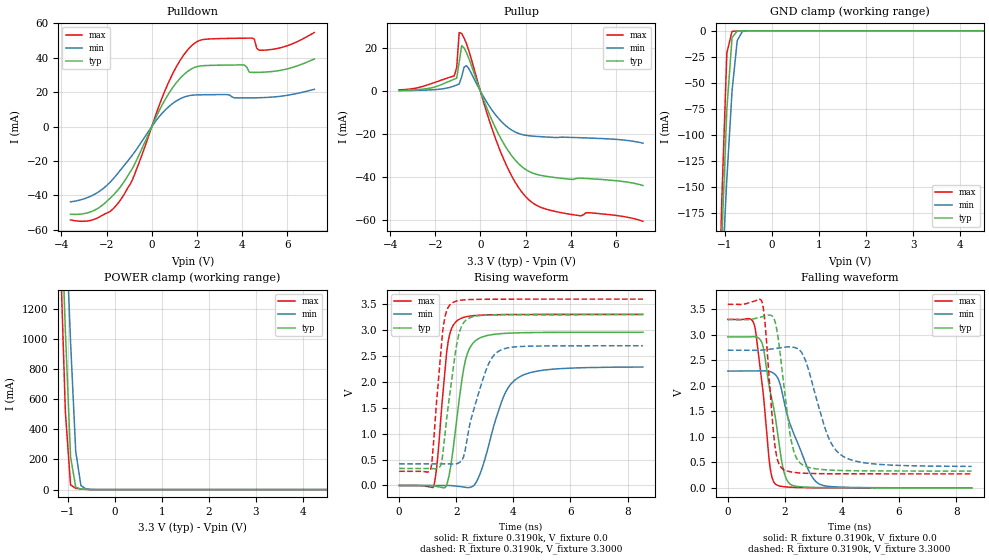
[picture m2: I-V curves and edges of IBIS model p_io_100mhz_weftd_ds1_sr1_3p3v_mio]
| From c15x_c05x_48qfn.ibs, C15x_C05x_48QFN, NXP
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[Model] p_io_100mhz_weftd_ds1_sr1_3p3v_mio
|   Model p_io_100mhz_weftd_ds1_sr1_3p3v_mio
| This model was characterised for following simulation conditions:
| External (pad) voltage:
|   - Typ: 3.3V,   - Min: 2.7V,   - Max: 3.6V
| Library cells for typ/min/max conditions are connected as defined below:
|  pad - External Pad
|  ipp_do_lv - Core Input
|  ipp_obe_lv - Output Buffer Enable
|  IOGC - NC
|  REFH3V3 - REFH3V3
|  REFL3V3 - REFL3V3
|  ZI - NC
|  abut_ncal_vddio[1] - vddio
|  abut_ncal_vddio[2] - vddio
|  abut_ncal_vddio[3] - vssio
|  abut_ncal_vddio[4] - vddio
|  abut_ncal_vddio[5] - vddio
|  abut_ncal_vddio[6] - vssio
|  abut_pcal_vddio[1] - vssio
|  abut_pcal_vddio[2] - vssio
|  abut_pcal_vddio[3] - vddio
|  abut_pcal_vddio[4] - vssio
|  abut_pcal_vddio[5] - vssio
|  abut_pcal_vddio[6] - vddio
|  ipp_do_1p8v - ipp_do_1p8v
|  ipp_dse_lv - vdd_lv
|  ipp_eftd_lv - NC
|  ipp_ina_mux_vddio - NC
|  ipp_ina_mux_vddio[0] - NC
|  ipp_ina_mux_vddio[1] - NC
|  ipp_ina_r0_vddio - NC
|  ipp_ina_r0a_vddio - NC
|  ipp_ina_r0b_vddio - NC
|  ipp_ina_r0c_vddio - NC
|  ipp_ina_r0d_vddio - NC
|  ipp_ina_r0e_vddio - NC
|  ipp_ina_r0f_vddio - NC
|  ipp_ina_r300_vddio - NC
|  ipp_ina_r300a_vddio - NC
|  ipp_ina_r300b_vddio - NC
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Model_type I/O
Polarity   Non-Inverting
Enable   Active-High
Vinl =   0.9900V
Vinh =   2.3100V
Vmeas =  1.6500V
Cref =   30.0000pF
Rref =   1.0000M
Vref =   3.3000V
C_comp   1.3824pF   1.3233pF   1.4661pF
|C_comp_pullup   0.6942pF   0.7256pF   0.6724pF
|C_comp_pulldown   0.6072pF   0.6599pF   0.5691pF
[Model Spec]
| variable   typ   min   max
Vinh   2.3100V   1.8900V   2.5200V
Vinl   0.9900V   0.8100V   1.0800V
[Temperature Range]   25.0000   0.1250k   -40.0000
[Voltage Range]   3.3000V   2.7000V   3.6000V
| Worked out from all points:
|   slope of the pulldown table from 0 to 0.495 V, typ, clamps not added: 36.8 ohm
|   slope of the pullup table from 0 to 0.495 V, typ, clamps not added: 37.8 ohm
|   GND clamp passes 1 mA (typ) near -0.75 V on its own axis
|   POWER clamp passes 1 mA (typ) near -0.55 V on its own axis
|   rising waveform, R_fixture 0.3190k, V_fixture 0.0: 20-80 % time 437ps typ, 779ps min, 310ps max; typ from 0 V to 2.96 V
|   rising waveform, R_fixture 0.3190k, V_fixture 3.3000: 20-80 % time 419ps typ, 681ps min, 295ps max; typ from 0.33 V to 3.3 V
|   falling waveform, R_fixture 0.3190k, V_fixture 0.0: 20-80 % time 516ps typ, 821ps min, 360ps max; typ from 2.96 V to 0 V
|   falling waveform, R_fixture 0.3190k, V_fixture 3.3000: 20-80 % time 404ps typ, 756ps min, 278ps max; typ from 3.3 V to 0.33 V
[Pulldown]
|Voltage   I(typ)   I(min)   I(max)
-3.6V     -50.99mA   -43.76mA   -54.26mA
-2.5V     -48.39mA   -39.11mA   -53.69mA
-1.4V     -35.22mA   -25.46mA   -42.92mA
-850mV    -24.19mA   -16.4mA    -30.69mA
800mV     20.23mA    12.14mA    27.32mA
1.35V     29.37mA    16.76mA    40.44mA
1.9V      34.45mA    18.38mA    48.57mA
4.1V      35.83mA    16.68mA    51.45mA
4.43V     31.54mA    16.72mA    51.52mA
4.65V     31.54mA    16.77mA    45.56mA
5.09V     31.78mA    16.98mA    44.58mA
7.2V      39.32mA    21.7mA     54.71mA
[Pullup]
|Voltage   I(typ)   I(min)   I(max)
-3.6V     392.3uA    235.2uA    607.2uA
-1.16V    5.571mA    2.41mA     7.094mA
-1.05V    6.017mA    2.857mA    10.99mA
-940mV    13.55mA    3.321mA    27.21mA
-830mV    21.12mA    6.673mA    26.77mA
-720mV    20.02mA    11.25mA    24.57mA
-610mV    17.72mA    11.8mA     21.82mA
820mV     -20.27mA   -12.85mA   -26.19mA
1.48V     -31.2mA    -18.62mA   -41.17mA
2.03V     -36.53mA   -20.52mA   -49.25mA
3.46V     -40.29mA   -21.47mA   -56.15mA
7.2V      -43.77mA   -24.12mA   -60.4mA
[GND_clamp]
|Voltage   I(typ)   I(min)   I(max)
-3.6V     -4.179A    -3.084A    -5.65A
-1.18V    -350.3mA   -344.8mA   -366.5mA
-1.07V    -203.5mA   -240.3mA   -165.6mA
-960mV    -75.17mA   -142.1mA   -21.27mA
-850mV    -6.53mA    -58.02mA   -538.4uA
-740mV    -289.9uA   -9.332mA   -209.1uA
-630mV    -85.04uA   -601.4uA   -92.54uA
-300mV    -199.1nA   -1.25uA    -48.79nA
7.2V      0A         0A         0A
[POWER_clamp]
|Voltage   I(typ)   I(min)   I(max)
-3.6V     24.55A     22.33A     26.93A
-1.16V    2.047A     2.721A     1.599A
-1.05V    1.052A     1.848A     514.6mA
-940mV    218.8mA    982.2mA    31.26mA
-830mV    15.16mA    252.6mA    8.517mA
-720mV    4.307mA    26.88mA    4.483mA
-610mV    1.728mA    3.641mA    1.672mA
7.2V      0A         0A         0A
[Ramp]
| variable   typ   min   max
dV/dt_r  1.7760/0.4370n   1.3734/0.7794n   1.9829/0.3103n
dV/dt_f  1.7821/0.4039n   1.3673/0.7561n   1.9953/0.2776n
R_load = 0.3190k
[Rising Waveform]
R_fixture= 0.3190k
V_fixture= 0.0
V_fixture_min= 0.0
V_fixture_max= 0.0
|time   V(typ)   V(min)   V(max)
0s        3.011nV    251.5nV    9.8nV
1.206ns   -7.522mV   -184.8uV   -19.52mV
1.335ns   -19.53mV   138.3uV    458.1mV
1.699ns   73.68mV    511.5uV    2.716V
2.066ns   1.506V     -15.7mV    3.197V
2.297ns   2.357V     -33.82mV   3.254V
2.579ns   2.744V     -16.26mV   3.279V
3.663ns   2.937V     1.724V     3.302V
4.159ns   2.949V     2.079V     3.304V
8.54ns    2.96V      2.289V     3.305V
[Rising Waveform]
R_fixture= 0.3190k
V_fixture= 3.3000
V_fixture_min= 2.7000
V_fixture_max= 3.6000
|time   V(typ)   V(min)   V(max)
0s        329.6mV    418.3mV    274.4mV
1.109ns   328.4mV    418.1mV    324.6mV
1.42ns    356.5mV    418.8mV    2.349V
1.532ns   621.3mV    419.3mV    3.006V
1.841ns   2.037V     415.3mV    3.519V
2.046ns   2.811V     426.2mV    3.569V
2.252ns   3.139V     548mV      3.585V
2.984ns   3.288V     2.134V     3.597V
3.493ns   3.295V     2.597V     3.599V
8.54ns    3.3V       2.7V       3.6V
[Falling Waveform]
R_fixture= 0.3190k
V_fixture= 0.0
V_fixture_min= 0.0
V_fixture_max= 0.0
|time   V(typ)   V(min)   V(max)
0s        2.96V      2.291V     3.305V
934.7ps   2.967V     2.29V      3.188V
1.227ns   2.791V     2.294V     1.925V
1.473ns   1.923V     2.283V     435.9mV
1.698ns   1.264V     2.2V       62.87mV
1.909ns   461.1mV    1.863V     26.49mV
2.107ns   120.5mV    1.382V     15.31mV
2.819ns   11.96mV    356.5mV    3.259mV
3.189ns   6.067mV    80.38mV    1.687mV
8.54ns    88.34uV    282uV      53.95uV
[Falling Waveform]
R_fixture= 0.3190k
V_fixture= 3.3000
V_fixture_min= 2.7000
V_fixture_max= 3.6000
|time   V(typ)   V(min)   V(max)
0s        3.3V       2.7V       3.6V
1.198ns   3.354V     2.701V     3.648V
1.316ns   3.371V     2.707V     3.169V
1.651ns   3.271V     2.732V     830.4mV
1.922ns   2.201V     2.753V     371.2mV
2.259ns   831.2mV    2.76V      308.2mV
2.651ns   441.4mV    2.59V      287.4mV
3.467ns   352.7mV    1.074V     277mV
4.001ns   339.9mV    632.4mV    275.6mV
8.54ns    329.9mV    421.2mV    274.5mV
